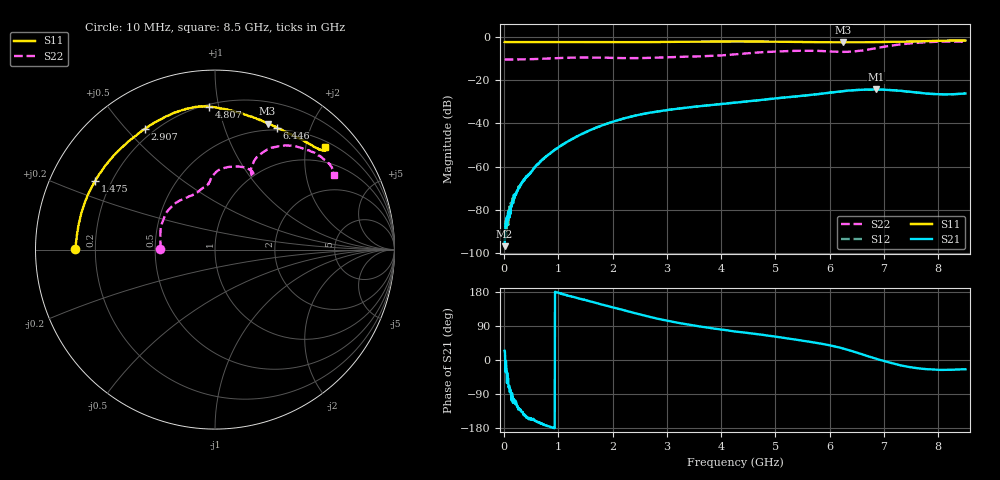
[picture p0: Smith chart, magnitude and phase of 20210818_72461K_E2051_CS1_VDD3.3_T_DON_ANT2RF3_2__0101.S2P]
!Agilent Technologies,E5071C,MY46417908,A.11.23
!Date: Wed Aug 18 14:30:33 2021
!Data & Calibration Information:
!Freq	S11:SOLT2(ON)	S21:SOLT2(ON)	S12:SOLT2(ON)	S22:SOLT2(ON)
!PortZ  Port1:50+j0  Port2:50+j0
!Above PortZ is port z conversion or system Z0 setting when saving the data.
!When reading, reference impedance value at option line is always used.
# Hz S dB R 50
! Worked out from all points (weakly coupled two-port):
!   1601 points, 10 MHz to 8.5 GHz, reference 50 ohm
!   highest |S21| = -24.22 dB at 6.86 GHz (marker M1); lowest = -97.0 dB at 10 MHz (marker M2)
!   lowest |S11| = -2.4 dB at 6.25 GHz (marker M3), VSWR 7.33, Z = 21.3 + j70.7 ohm
!   |S11| at or under -10 dB: nowhere
!   |S22| runs from -10.3 to -2.0 dB; largest |S21 - S12| = 0.00029
!   S11 on the Smith chart (normalised r, x): 10 MHz: 0.12, +0.00; 1.475 GHz: 0.14, +0.26; 2.907 GHz: 0.17, +0.56; 4.807 GHz: 0.22, +0.94; 6.446 GHz: 0.47, +1.52; 8.5 GHz: 0.63, +2.41
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1e7  -2.16 179.7  -96.95 24.7  -92.89 51.5  -10.30 179.6
6.836875e7  -2.20 178.5  -84.67 -59.9  -82.67 -72.3  -10.32 178.3
1.055125e8  -2.20 177.7  -83.57 -84.8  -79.43 -76.3  -10.33 177.4
2.169438e8  -2.23 175.4  -72.44 -111.9  -73.19 -110.7  -10.32 174.7
3.28375e8  -2.23 173.2  -67.49 -136.5  -67.85 -132.1  -10.26 172.4
6.149125e8  -2.25 167.3  -59.14 -163.6  -58.96 -164.0  -10.05 165.4
9.810438e8  -2.26 159.9  -51.47 178.2  -51.45 178.4  -9.65 154.3
1.426769e9  -2.27 151.0  -44.96 160.8  -45.04 161.0  -9.36 139.3
1.474525e9  -2.28 150.0  -44.40 158.8  -44.41 158.9  -9.36 137.7
2.137806e9  -2.27 136.3  -38.19 134.0  -38.18 134.0  -9.64 118.4
2.843538e9  -2.19 121.3  -34.36 108.5  -34.35 108.4  -9.42 105.6
2.907212e9  -2.18 120.1  -34.16 106.7  -34.16 106.6  -9.35 104.7
4.255e9  -1.93 98.8  -30.33 75.3  -30.33 75.3  -7.92 92.7
4.80685e9  -1.98 92.3  -28.87 65.6  -28.87 65.6  -6.87 84.9
5.671769e9  -2.23 78.9  -26.69 47.2  -26.70 47.3  -6.28 66.4
6.25015e9  -2.38 67.3  -25.01 30.1  -25.02 30.0  -6.77 62.9
6.446481e9  -2.37 63.2  -24.55 21.8  -24.57 21.6  -6.56 64.6
6.860369e9  -2.24 55.0  -24.22 3.1  -24.24 3.0  -5.01 65.8
7.088538e9  -2.13 51.1  -24.45 -6.3  -24.47 -6.5  -4.04 62.4
7.497119e9  -1.98 45.6  -25.36 -19.2  -25.36 -19.4  -2.81 52.9
8.001212e9  -1.65 42.0  -26.41 -25.9  -26.38 -25.9  -2.07 39.6
8.5e9  -1.53 42.9  -26.09 -24.3  -26.07 -24.6  -2.15 32.1
